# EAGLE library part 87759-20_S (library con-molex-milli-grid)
HEADER
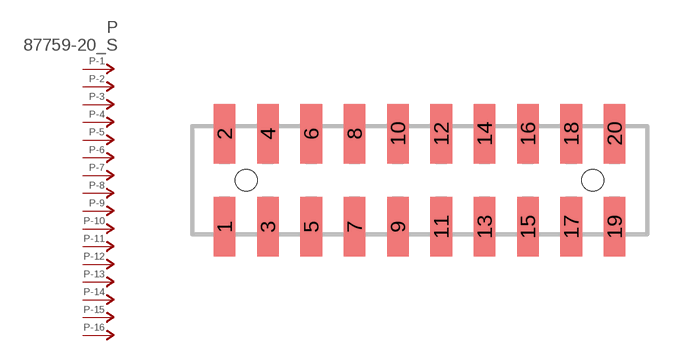
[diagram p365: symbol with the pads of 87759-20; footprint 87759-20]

Designator prefix P; gates -1=P-NV -2=P-N -3=P-N -4=P-N -5=P-N -6=P-N -7=P-N -8=P-N -9=P-N -10=P-N -11=P-N -12=P-N -13=P-N -14=P-N -15=P-N -16=P-N -17=P-N -18=P-N -19=P-N -20=P-N

## 87759-20_S  [87759-20]
1  -1:P  pas
2  -2:P  pas
3  -3:P  pas
4  -4:P  pas
5  -5:P  pas
6  -6:P  pas
7  -7:P  pas
8  -8:P  pas
9  -9:P  pas
10  -10:P  pas
11  -11:P  pas
12  -12:P  pas
13  -13:P  pas
14  -14:P  pas
15  -15:P  pas
16  -16:P  pas
17  -17:P  pas
18  -18:P  pas
19  -19:P  pas
20  -20:P  pas

## Footprint 87759-20 (pad centres in mm)
HEADER SMD Dual Row, Vertical
smd 1 x 2.75: 1 -9,-2.15; 2 -9,2.15; 3 -7,-2.15; 4 -7,2.15; 5 -5,-2.15; 6 -5,2.15; 7 -3,-2.15; 8 -3,2.15; 9 -1,-2.15; 10 -1,2.15; 11 1,-2.15; 12 1,2.15; 13 3,-2.15; 14 3,2.15; 15 5,-2.15; 16 5,2.15; 17 7,-2.15; 18 7,2.15; 19 9,-2.15; 20 9,2.15
hole 1 at -8,0
hole 1 at 8,0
